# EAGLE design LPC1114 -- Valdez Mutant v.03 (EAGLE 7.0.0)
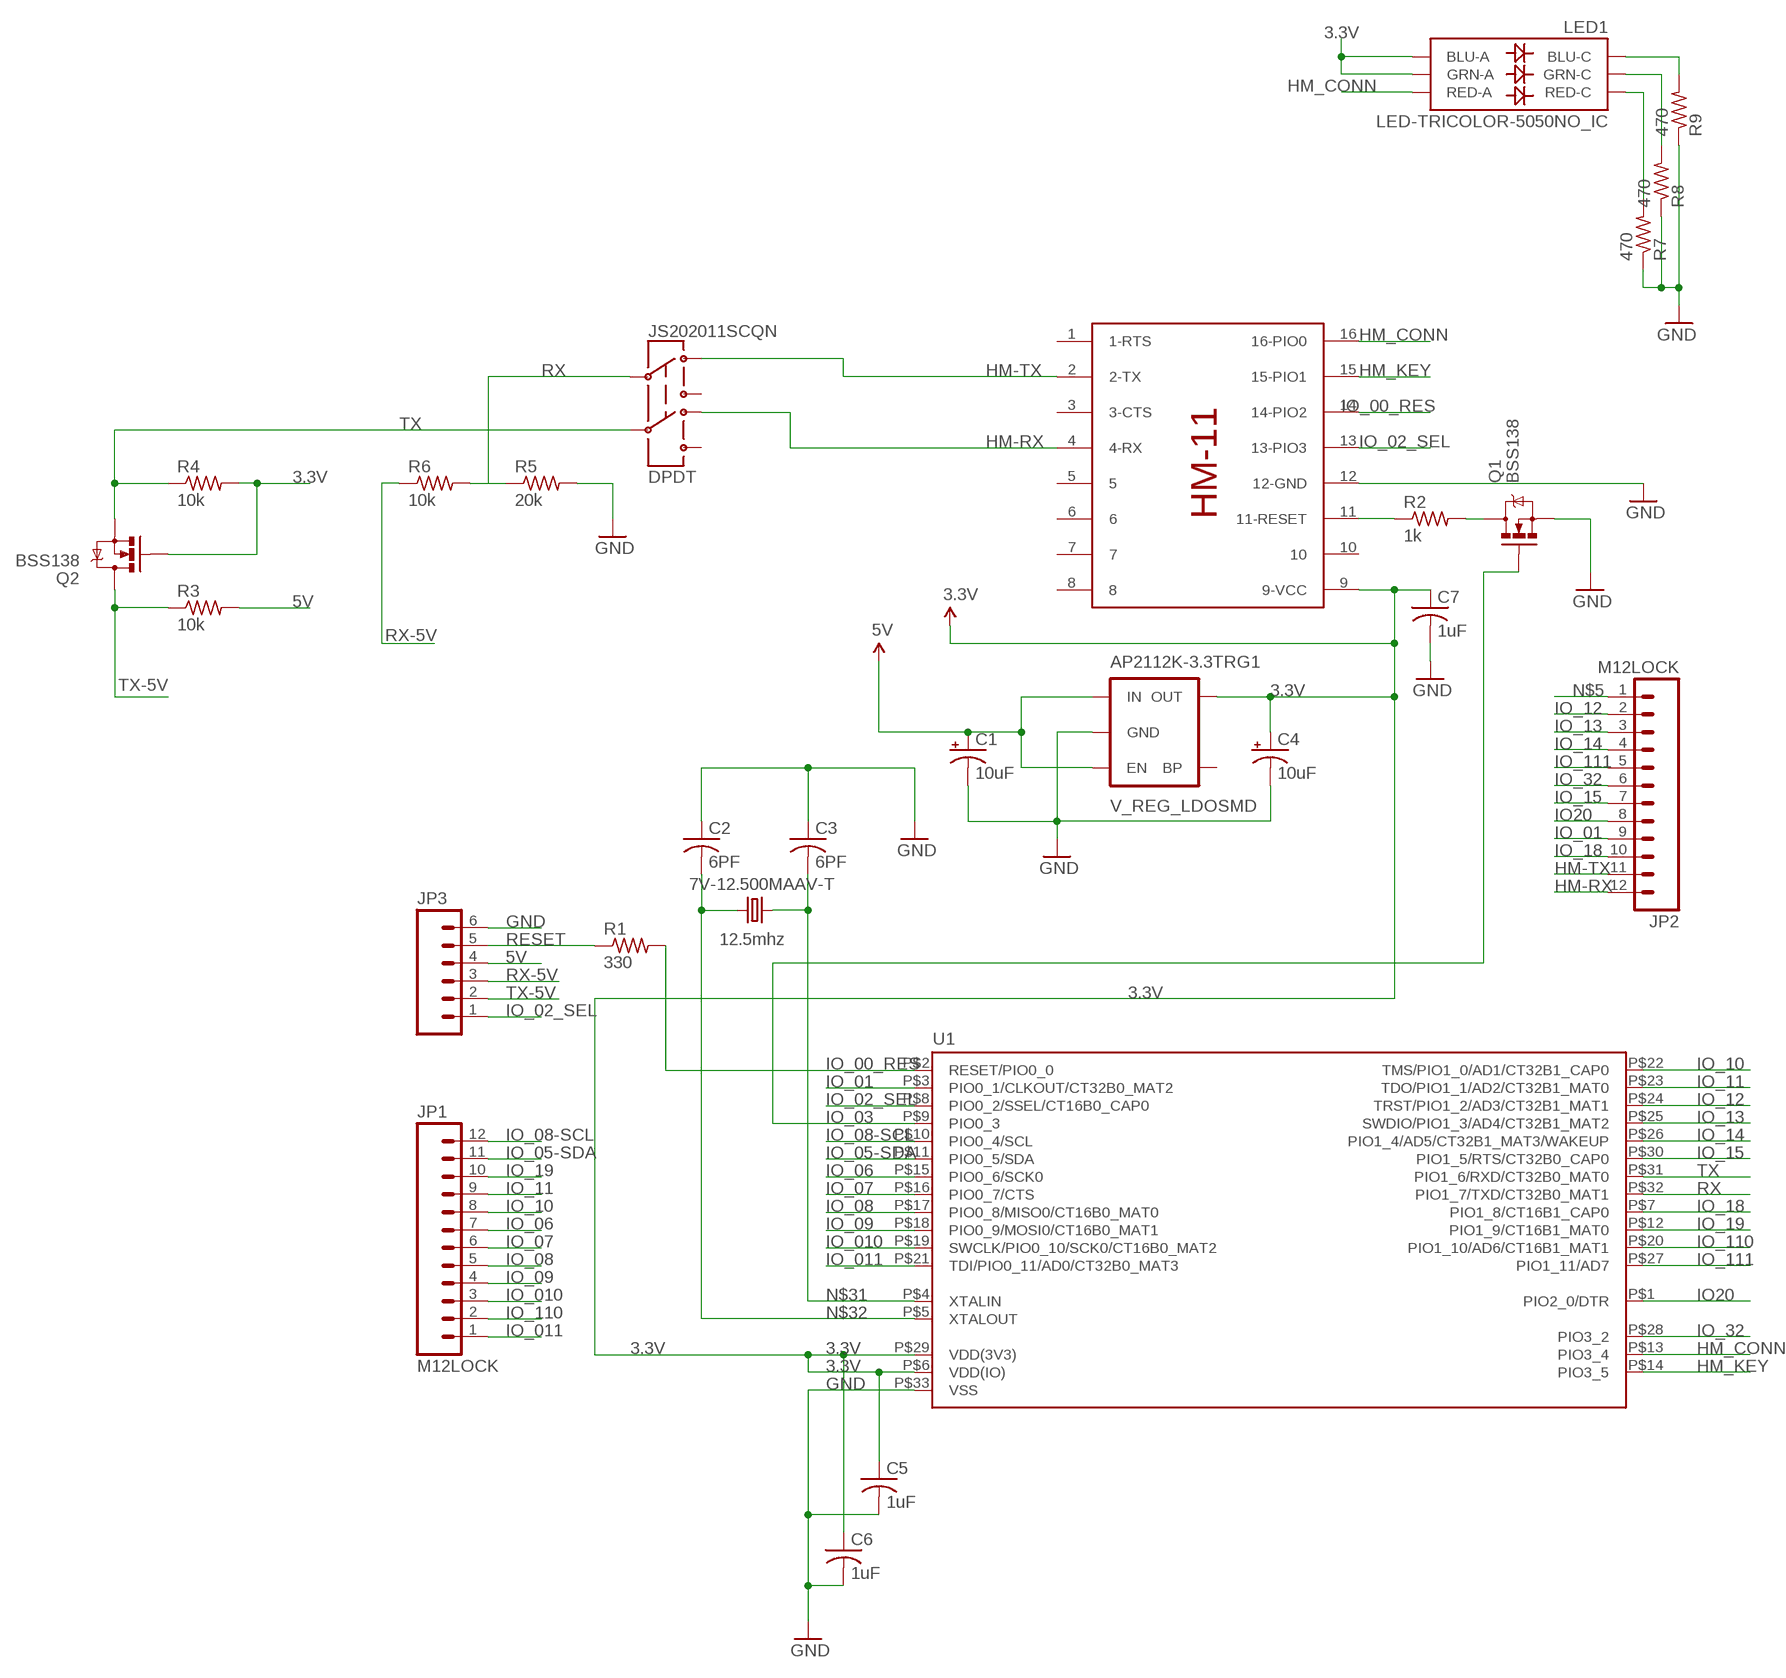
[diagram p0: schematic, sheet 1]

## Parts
7V-12.500MAAV-T  12.5mhz  CRYSTAL5X3  [CRYSTAL-SMD-5X3]
AP2112K-3.3TRG1  V_REG_LDOSMD  [SOT23-5]
C1  10uF  CAP_POL1206  [EIA3216]
C2  6PF  C-USC0402K  [C0402K]
C3  6PF  C-USC0402K  [C0402K]
C4  10uF  CAP_POL1206  [EIA3216]
C5  1uF  C-USC0402K  [C0402K]
C6  1uF  C-USC0402K  [C0402K]
C7  1uF  C-USC0402K  [C0402K]
JP1  M12LOCK  [1X12_LOCK]
JP2  M12LOCK  [1X12_LOCK]
JP3  M06LOCK  [1X06_LOCK]
JS202011SCQN  DPDT  SWITCH-DPDTAYZ0202  [AYZ0202]
LED1  LED-TRICOLOR-5050NO_IC  [LED-TRICOLOR-5050]
Q1  BSS138  MOSFET-NCHANNELBSS138  [SOT23]
Q2  BSS138  MOSFET-NCHANNELBSS138  [SOT23]
R1  330  R-US_R0402  [R0402]
R2  1k  R-US_R0402  [R0402]
R3  10k  R-US_R0402  [R0402]
R4  10k  R-US_R0402  [R0402]
R5  20k  R-US_R0402  [R0402]
R6  10k  R-US_R0402  [R0402]
R7  470  R-US_R0402  [R0402]
R8  470  R-US_R0402  [R0402]
R9  470  R-US_R0402  [R0402]
U1  LPC1113/4_QFN  [HVQFN33-7X7]
U$1  HM-11  [HM-11]

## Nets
3.3V: AP2112K-3.3TRG1.5(OUT) C4.A(+) C5.1 C6.1 C7.1 LED1.1(GRN-A) LED1.3(BLU-A) Q2.1(G) R4.2 U1.P$6(VDD(IO)) U1.P$29(VDD(3V3)) U$1.9(9-VCC)
5V: AP2112K-3.3TRG1.1(IN) AP2112K-3.3TRG1.3(EN) C1.A(+) JP3.4 R3.2
GND: AP2112K-3.3TRG1.2(GND) C1.C(-) C2.1 C3.1 C4.C(-) C5.2 C6.2 C7.2 JP3.6 Q1.2(S) R5.2 R7.1 R8.1 R9.1 U1.P$33(VSS) U$1.12(12-GND)
HM-RX: JP2.12 JS202011SCQN.4 U$1.4(4-RX)
HM-TX: JP2.11 JS202011SCQN.1 U$1.2(2-TX)
HM_CONN: LED1.2(RED-A) U1.P$13(PIO3_4) U$1.16(16-PIO0)
HM_KEY: U1.P$14(PIO3_5) U$1.15(15-PIO1)
IO20: JP2.8 U1.P$1(PIO2_0/DTR)
IO_00_RES: R1.2 U1.P$2(RESET/PIO0_0) U$1.14(14-PIO2)
IO_01: JP2.9 U1.P$3(PIO0_1/CLKOUT/CT32B0_MAT2)
IO_02_SEL: JP3.1 U1.P$8(PIO0_2/SSEL/CT16B0_CAP0) U$1.13(13-PIO3)
IO_03: Q1.1(G) U1.P$9(PIO0_3)
IO_05-SDA: JP1.11 U1.P$11(PIO0_5/SDA)
IO_06: JP1.7 U1.P$15(PIO0_6/SCK0)
IO_07: JP1.6 U1.P$16(PIO0_7/CTS)
IO_08: JP1.5 U1.P$17(PIO0_8/MISO0/CT16B0_MAT0)
IO_08-SCL: JP1.12 U1.P$10(PIO0_4/SCL)
IO_09: JP1.4 U1.P$18(PIO0_9/MOSI0/CT16B0_MAT1)
IO_10: JP1.8 U1.P$22(TMS/PIO1_0/AD1/CT32B1_CAP0)
IO_010: JP1.3 U1.P$19(SWCLK/PIO0_10/SCK0/CT16B0_MAT2)
IO_11: JP1.9 U1.P$23(TDO/PIO1_1/AD2/CT32B1_MAT0)
IO_011: JP1.1 U1.P$21(TDI/PIO0_11/AD0/CT32B0_MAT3)
IO_12: JP2.2 U1.P$24(TRST/PIO1_2/AD3/CT32B1_MAT1)
IO_13: JP2.3 U1.P$25(SWDIO/PIO1_3/AD4/CT32B1_MAT2)
IO_14: JP2.4 U1.P$26(PIO1_4/AD5/CT32B1_MAT3/WAKEUP)
IO_15: JP2.7 U1.P$30(PIO1_5/RTS/CT32B0_CAP0)
IO_18: JP2.10 U1.P$7(PIO1_8/CT16B1_CAP0)
IO_19: JP1.10 U1.P$12(PIO1_9/CT16B1_MAT0)
IO_32: JP2.6 U1.P$28(PIO3_2)
IO_110: JP1.2 U1.P$20(PIO1_10/AD6/CT16B1_MAT1)
IO_111: JP2.5 U1.P$27(PIO1_11/AD7)
N$2: LED1.4(BLU-C) R9.2
N$3: LED1.6(GRN-C) R8.2
N$4: LED1.5(RED-C) R7.2
N$5: JP2.1
N$8: Q1.3(D) R2.2
N$9: R2.1 U$1.11(11-RESET)
N$31: 7V-12.500MAAV-T.3 C3.2 U1.P$4(XTALIN)
N$32: 7V-12.500MAAV-T.1 C2.2 U1.P$5(XTALOUT)
RESET: JP3.5 R1.1
RX: JS202011SCQN.2 R5.1 R6.2 U1.P$32(PIO1_7/TXD/CT32B0_MAT1)
RX-5V: JP3.3 R6.1
TX: JS202011SCQN.5 Q2.2(S) R4.1 U1.P$31(PIO1_6/RXD/CT32B0_MAT0)
TX-5V: JP3.2 Q2.3(D) R3.1
Unconnected: AP2112K-3.3TRG1.4(BP) JS202011SCQN.3 JS202011SCQN.6 U$1.1(1-RTS) U$1.3(3-CTS) U$1.5 U$1.6 U$1.7 U$1.8 U$1.10

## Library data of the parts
7V-12.500MAAV-T = SparkFun-FreqCtrl:CRYSTAL: Various standard crystals. Proven footprints. Spark Fun Electronics SKU : COM-00534
AP2112K-3.3TRG1 = SparkFun-PowerIC:V_REG_LDO: Voltage Regulator LDO Standard 150mA LDO voltage regulator in SOT-23 layout. Micrel part MIC5205. BP (by-pass) pin is used to lower output noise with 470pF cap.
C1 C4 = SparkFun-Capacitors:CAP_POL: Capacitor Polarized
C2 C3 C5-C7 = resistor:C-US: CAPACITOR, American symbol
JP1 JP2 = SparkFun-Connectors:M12: Header 12 Standard 12-pin 0.1" header. Use with straight break away headers (SKU : PRT-00116), right angle break away headers (PRT-00553), swiss pins (PRT-00743), machine pins (PRT-00117), and female headers (PRT-00115).
JP3 = SparkFun-Connectors:M06: Header 6 Standard 6-pin 0.1" header. Use with straight break away headers (SKU : PRT-00116), right angle break away headers (PRT-00553), swiss pins (PRT-00743), machine pins (PRT-00117), and female headers (PRT-00115). Molex polarized connector foot print use with SKU : PRT-08094 with associated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
JS202011SCQN = SparkFun-Electromechanical:SWITCH-DPDT: DPDT Version of the COM-00597; PROD_ID: SWCH-08179
LED1 = SparkFun-LED:LED-TRICOLOR-5050
Q1 Q2 = SparkFun-DiscreteSemi:MOSFET-NCHANNEL: Common NMOSFET Parts MFG P/NStore IDProd ID FDD8780TRANS-09984 SI7820DNTRANS-11055 FDS6630AIC-08089 2N7002PWTRANS-11151 FQP30N06L COM-10213TRANS-10060 BSS123LT1GTRANS-08345 BSS138TRANS-00830 BS170 2N7000; PROD_ID: TRANS-00830
R1-R9 = resistor:R-US_: RESISTOR, American symbol
U1 = microbuilder:LPC1113/4_QFN: LPC1113/4 ARM Cortex-M0 processor, running at frequencies of up to 50 MHz. QFN 33 Pin Package; DIGIKEY#: 568-4948-ND; MANF: NXP; MANF#: LPC1114FHN33/301,5
U$1 = HM-11:HM-11

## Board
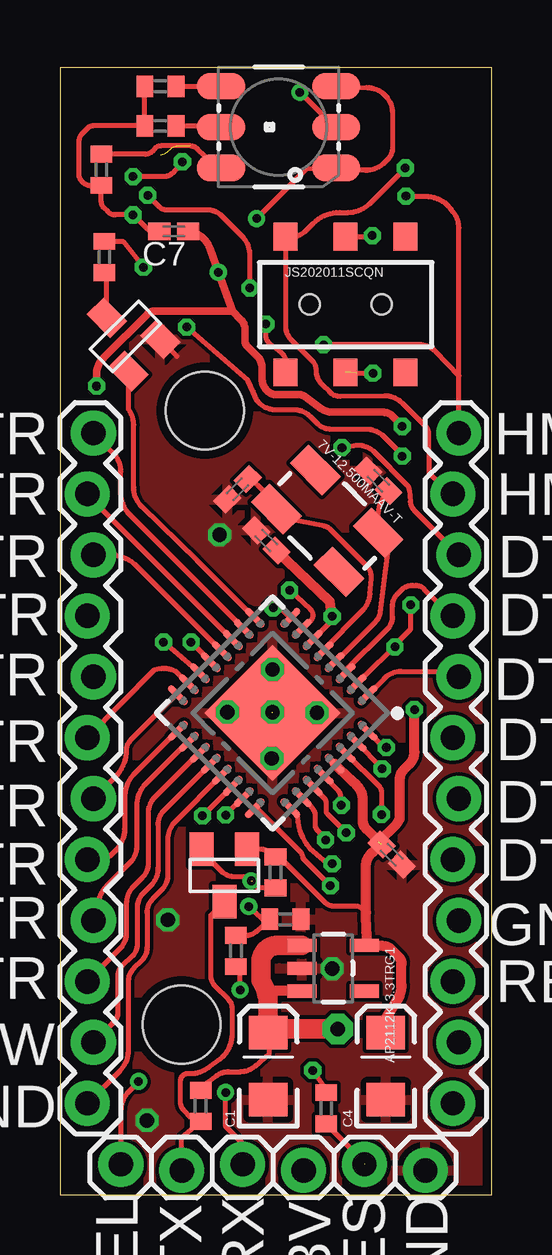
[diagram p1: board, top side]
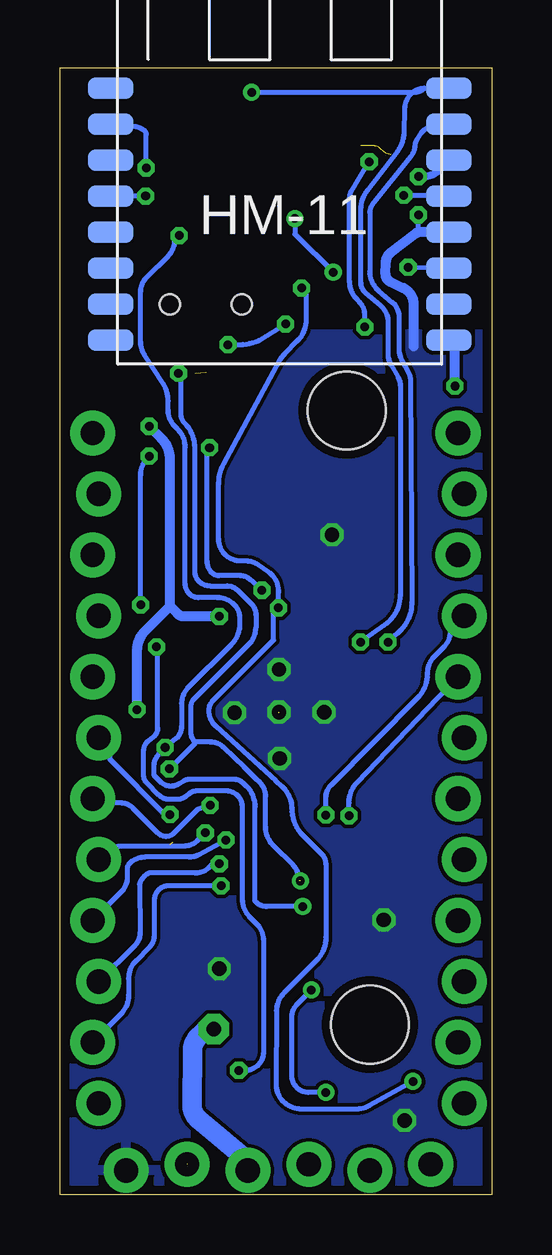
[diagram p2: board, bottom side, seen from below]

Size 18 x 46.97 mm. Coordinates in mm from the lower left corner, seen from the top.
Outline: 0,0 18,0 18,46.97 0,46.97 0,0
Copper layers (1*16): Top 0.0356mm / dielectric 1.5011mm / Bottom 0.0356mm
Design rules "LaenPCBOrder": minimum track width 6mil, minimum drill 13mil, track to track 6mil, track to pad 6mil, pad to pad 6mil, via to via 6mil, smd to smd 6mil, copper to edge 15mil, drill to drill 6mil, minimum pad ring 7mil, minimum via ring 7mil, stop-mask expansion 3mil, vias tented up to drill 0mil, thermal gap 10mil
Holes 3.25 mm at 5.07,7.1 6.04,32.68

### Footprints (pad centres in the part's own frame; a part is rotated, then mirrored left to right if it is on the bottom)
CRYSTAL-SMD-5X3 = smd 1.9 x 1.1: 1 -1.85,-1.15; 2 1.85,-1.15; 3 1.85,1.15; 4 -1.85,1.15
SOT23-5 = smd 0.55 x 1.2: 1 -0.95,-1.3; 2 0,-1.3; 3 0.95,-1.3; 4 0.95,1.3; 5 -0.95,1.3
EIA3216 = smd 1.4 x 1.6: A 1.4,0; C -1.4,0
C0402K = smd 0.925 x 0.74: 1 -0.6,0; 2 0.6,0
1X12_LOCK = drill 1.016 pad 1.88: 1 0,0.127; 2 2.54,-0.127; 3 5.08,0.127; 4 7.62,-0.127; 5 10.16,0.127; 6 12.7,-0.127; 7 15.24,0.127; 8 17.78,-0.127; 9 20.32,0.127; 10 22.86,-0.127; 11 25.4,0.127; 12 27.94,-0.127
1X06_LOCK = drill 1.016 pad 1.88: 1 0,0; 2 2.54,-0.254; 3 5.08,0; 4 7.62,-0.254; 5 10.16,0; 6 12.7,-0.254
AYZ0202 = smd 1 x 1.15: 1 -2.5,2.825; 2 0,2.825; 3 2.5,2.825; 4 -2.5,-2.825; 5 0,-2.825; 6 2.5,-2.825 | hole 0.85: 1.5,0; -1.5,0
LED-TRICOLOR-5050 = smd 2 x 1.1: 1 -2.4,1.7; 2 -2.4,0; 3 -2.4,-1.7; 4 2.4,-1.7; 5 2.4,0; 6 2.4,1.7
SOT23 = smd 1 x 1.4: 1 -0.95,-1.1; 2 0.95,-1.1; 3 0,1.1
R0402 = smd 0.7 x 0.9: 1 -0.65,0; 2 0.65,0
HVQFN33-7X7 = smd 1.067 x 0.3: P$1 -3.327,2.275; P$2 -3.327,1.625; P$3 -3.327,0.975; P$4 -3.327,0.325; P$5 -3.327,-0.325; P$6 -3.327,-0.975; P$7 -3.327,-1.625; P$8 -3.327,-2.275; P$17 3.327,-2.275; P$18 3.327,-1.625; P$19 3.327,-0.975; P$20 3.327,-0.325; P$21 3.327,0.325; P$22 3.327,0.975; P$23 3.327,1.625; P$24 3.327,2.275 | smd 0.3 x 1.067: P$9 -2.275,-3.327; P$10 -1.625,-3.327; P$11 -0.975,-3.327; P$12 -0.325,-3.327; P$13 0.325,-3.327; P$14 0.975,-3.327; P$15 1.625,-3.327; P$16 2.275,-3.327; P$25 2.275,3.327; P$26 1.625,3.327; P$27 0.975,3.327; P$28 0.325,3.327; P$29 -0.325,3.327; P$30 -0.975,3.327; P$31 -1.625,3.327; P$32 -2.275,3.327 | smd 4 x 4: P$33 0,0
HM-11 = smd 1.9 x 0.9: 1 -0.3,11.5; 2 -0.3,10; 3 -0.3,8.5; 4 -0.3,7; 5 -0.3,5.5; 6 -0.3,4; 7 -0.3,2.5; 8 -0.3,1; 9 13.8,1; 10 13.8,2.5; 11 13.8,4; 12 13.8,5.5; 13 13.8,7; 14 13.8,8.5; 15 13.8,10; 16 13.8,11.5

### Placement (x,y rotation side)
7V-12.500MAAV-T  11.15,28.09 315 top
AP2112K-3.3TRG1  11.4,9.44 270 top
C1  8.69,5.36 90 top
C2  7.4,29.41 45 top
C3  13.28,29.75 315 top
C4  13.59,5.36 90 top
C5  13.84,14.18 315 top
C6  8.61,27.27 135 top
C7  4.75,40.16 180 top
JP1  1.27,3.81 90 top
JP2  16.51,3.81 90 top
JP3  2.54,1.27 0 top
JS202011SCQN  11.91,37.11 0 top
LED1  9.12,44.5 180 top
Q1  2.73,35.78 45 top
Q2  6.86,13.31 180 top
R1  11.1,3.61 90 top
R2  1.85,39.09 270 top
R3  5.87,3.71 90 top
R4  8.99,13.44 90 top
R5  9.4,11.48 0 top
R6  7.34,10.16 90 top
R7  4.19,44.55 0 top
R8  1.73,42.72 90 top
R9  4.19,46.2 0 top
U1  8.87,20.08 225 top
U$1  15.59,34.62 0 bottom

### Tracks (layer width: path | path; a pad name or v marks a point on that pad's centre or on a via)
3.3V  (via drill 0.36, 0.36 pad 0.25)  (1 unrouted)
  Top 0.203: AP2112K-3.3TRG1.5 | 11.35,23.94 U1.P$6 | Q2.1 8.33,14.41 arc-45 8.91,14.17 R4.2 9.15,14.09 11.08,12.16 arc45 11.37,12.04 12.3,12.04 arc-45 12.62,11.9 12.77,11.76 | LED1.3 12.79,46.15 arc-90 13.87,45.07 13.87,43.64 arc-45 13.67,43.16 13.53,43.02 arc-45 12.75,42.7 12.08,42.7 LED1.1 10.26,42.75 v8.2,40.69 | v6.6,38.46 6.6,38.44 6.62,38.42
  Top 0.305: v14.28,32.03 13.86,32.46 arc46 13.5,32.61 11.37,32.61 arc-37 10.88,32.78 10.21,33.27 arc37 9.98,33.35 9,33.35 arc-45 8.68,33.48 8.64,33.52 arc-45 8.43,34.02 8.43,34.44 arc45 8.22,34.96 7.81,35.37 arc-45 7.72,35.58 7.72,36.06 arc45 7.55,36.46 7.19,36.83 | v1.52,33.71 1.52,34.16 arc-45 1.83,34.91 3.62,36.7 arc-45 3.95,36.83 7.19,36.83 | 7.19,36.83 6.62,38.42 6.27,39.43 arc64 C7.1
  Top 0.406: U1.P$29 12.14,17.3 12.38,17.05 arc-45 12.62,16.48 12.62,15.6 arc45 12.77,15.24 C5.1 13.01,14.25 12.98,14.22 arc45 12.75,13.68 12.77,11.76 12.78,10.95 12.78,10.47 AP2112K-3.3TRG1.5 12.73,10.36 13.48,10.36 arc-45 13.84,10.22 14.11,9.95 arc-45 14.25,9.61 14.25,8.75 arc-31 14.07,8.12 13.61,7.37 C4.A | v14.78,20.22 14.78,18.45 arc-45 14.58,17.95 14.34,17.72 arc45 14.17,17.31 14.17,15.78 arc-45 14.04,15.47 13.28,14.71 | 11.35,23.94 v11.35,24.11 11.25,24.73 C6.1
  Bottom 0.203: v8.2,40.69 8.2,40.02 8.17,40.02 v6.6,38.46
  Bottom 0.406: v14.78,20.22 14.78,22.67 arc45 14.43,23.52 13.41,24.54 | 13.41,24.54 13.41,30.67 arc-45 13.76,31.52 v14.28,32.03 | v1.52,33.71 1.52,35.36 U$1.9 | 11.23,23.98 v11.35,24.11 12.81,24.11 arc45 13.1,24.23 13.41,24.54
5V  (via drill 0.6 pad 1.27)
  Top 0.203: AP2112K-3.3TRG1.3 | 8.84,6.91 C1.A 8.74,6.71 8.74,5.89 8.13,5.36 arc-41 7.53,5.13 7.05,5.13 arc37 6.53,4.96 5.93,4.51 R3.2
  Top 0.406: 8.59,8.51 9.68,8.51 AP2112K-3.3TRG1.3
  Top 0.813: 8.77,6.68 C1.A 8.69,8.1 arc17 8.66,8.25 8.59,8.51 8.38,8.94 8.38,9.68 arc-45 8.6,10.2 arc-45 9.06,10.39 AP2112K-3.3TRG1.1 | v11.58,6.91 8.84,6.91
  Bottom 0.813: JP3.4 10.16,1.42 12.18,3.09 arc51 12.49,3.76 12.47,5.97 arc45 12.2,6.62 11.91,6.91 v11.58,6.91
GND  (via drill 0.36, 0.6 pad 0.81)  (1 unrouted)
  Top 0.203: 4.15,40.11 C7.2 3.94,40.16 arc-45 3.58,40.31 v3.05,40.84 2.31,40.84 arc-45 2.01,40.97 1.83,41.15 arc-45 1.73,41.39 R8.1 1.72,42.06 1.3,42.06 arc-45 0.94,42.21 0.9,42.25 arc-45 0.79,42.53 0.79,43.87 arc-45 0.94,44.25 1.16,44.47 arc-45 1.37,44.55 R7.1 | Q1.2 4.18,35.64 4.88,34.95 | 3.54,44.53 R7.1 | R7.1 R9.1
  Bottom 0.203: 3.06,40.12 3.06,40.42 v3.05,40.84
  Bottom 0.406: 3.25,35.36 3.25,37.13 arc-64 3.67,37.79 4.23,38.06 arc64 4.42,38.36 4.41,38.88 arc51 4.21,39.26 3.17,40.07 arc25 3.06,40.12 U$1.12
  other vias: 8.86,20.12 8.86,21.89 10.72,20.09 8.84,18.19 6.99,20.12 3.63,3.1 11.35,9.42 4.5,11.46 6.65,27.51
  pour Bottom: 0,35.86 0,0 17.78,0 17.78,35.86
  pour Top: 0.2,36.07 0,0 17.78,0 17.98,36.07
HM-RX  (via drill 0.36, 0.36 pad 0.25)
  Top 0.203: JS202011SCQN.4 9.41,34.72 arc52 9.22,35.11 8.72,35.51 arc-18 8.66,35.57 8.66,35.57 arc-34 8.59,35.82 v8.59,36.3 | JP2.12 16.64,34.14 | 16.64,34.14 16.64,40.3 arc38 16.41,40.95 16.3,41.09 arc52 15.25,41.6 14.45,41.6 v14.43,41.63 | 16.64,34.14 15.68,35.14 arc46 14.98,35.43 v11,35.43
  Bottom 0.203: v14.43,41.63 15.88,41.63 U$1.4 | v11,35.43 10.5,35.43 arc-25 9.7,35.61 v8.59,36.3
HM-TX  (via drill 0.36 pad 0.25)
  Top 0.203: v14.4,42.8 12.92,41.32 arc-45 12.02,40.95 11.66,40.95 arc45 10.57,40.49 10.27,40.19 arc-45 9.65,39.93 JS202011SCQN.1 9.42,39.92 9.42,36.17 arc45 9.64,35.65 10.52,34.77 arc-45 10.69,34.35 arc45 10.93,33.77 11.25,33.45 arc46 11.68,33.28 13.54,33.3 arc-45 14.28,33 15.25,32.05 arc-45 15.37,31.76 15.39,30.07 JP2.11
  Bottom 0.203: v14.4,42.8 14.4,44.2 arc-45 14.45,44.32 arc-45 14.94,44.53 15.79,44.53 U$1.2
HM_CONN  (via drill 0.36, 0.36 pad 0.25)
  Top 0.203: U1.P$13 6.22,22.2 6.22,22.28 v5.46,23.04 | LED1.2 11.51,44.45 v10.01,45.95
  Bottom 0.203: 2.81,46.12 arc-54 3.43,45.81 arc-34 3.62,45.27 3.65,44.26 arc36 3.91,43.51 5.18,41.86 arc-37 5.46,41.09 5.46,38.03 arc-50 5.26,37.6 4.64,37.08 arc50 4.32,36.38 4.32,35.03 arc-30 4.21,34.6 3.89,34.06 arc30 3.81,33.74 3.81,25.02 arc55 4.47,23.74 v5.46,23.04 | 2.81,46.12 U$1.16 | v10.01,45.95 3.24,45.95 arc-45 2.81,46.12
HM_KEY  (via drill 0.36 pad 0.25)
  Top 0.203: U1.P$14 5.83,21.76 v4.32,23.04
  Bottom 0.203: U$1.15 1.86,44.55 2.34,44.55 arc-57 2.96,44.22 3.1,44 arc-30 3.18,43.76 arc35 3.37,43.27 4.97,41.26 arc-39 5.08,40.95 5.08,38.48 arc-49 4.71,37.69 4.13,37.19 arc49 3.86,36.6 3.86,35.25 arc-28 3.74,34.78 3.46,34.26 arc28 3.38,33.95 3.33,24.67 arc48 3.88,23.43 v4.32,23.04
IO20
  Top 0.203: U1.P$1 13.53,21.53 arc-45 14.23,21.82 16.41,21.82 JP2.8
IO_00_RES  (via drill 0.36, 0.36 pad 0.25)
  Top 0.203: 12.37,21.31 U1.P$2 13.11,22.02 v13.97,22.84 13.97,22.91 14.59,23.53 arc45 14.63,23.62 v14.63,24.59 | v14.28,30.79 14.22,30.89 13.5,31.61 arc45 12.79,31.9 11.33,31.9 arc-45 10.72,32.16 10.45,32.43 arc45 9.76,32.72 8.95,32.72 arc-48 8.22,33.1 8.05,33.49 7.84,33.94 v5.28,36.17 5.54,36.17 | v5.11,43.05 4.69,42.58 arc-44 4.35,42.44 v3.05,42.44 | 11.19,4.31 R1.2 11.1,4.42 v10.54,5.18
  Bottom 0.203: v13.97,22.84 13.92,22.78 13.92,19.44 arc52 14.09,19.09 14.33,18.91 arc-52 14.5,18.55 14.5,17.43 arc-45 14.41,17.2 13.86,16.65 arc-45 13.46,16.48 13.09,16.48 arc-41 12.72,16.62 12.64,16.69 arc41 12.25,16.84 11.09,16.84 arc49 10.56,16.6 arc41 10.39,16.15 10.39,12.32 arc-45 10.08,11.58 9.8,11.3 arc45 9.5,10.58 9.5,5.94 arc54 9.81,5.34 arc36 10.31,5.18 v10.54,5.18 | v14.63,24.59 14.63,30.01 arc49 v14.28,30.79 | v5.28,36.17 5.28,36.66 arc-45 5.51,37.21 5.6,37.3 arc45 5.92,38.06 5.92,41.56 arc27 5.85,41.83 v5.11,43.05
  Bottom 0.305: v3.05,42.44 2.82,42.44 arc-45 2.22,42.69 U$1.14
IO_01
  Top 0.203: U1.P$3 11.91,21.84 13.68,23.61 arc45 13.87,24.07 13.87,24.52 arc-45 14.1,25.07 14.23,25.21 arc-45 14.7,25.4 14.83,25.4 arc-45 15.19,25.25 15.65,24.79 16.26,24.21 JP2.9
IO_02_SEL  (via drill 0.36, 0.36 pad 0.25)
  Top 0.203: v8.89,24.46 9.3,24.36 U1.P$8 | v7.92,37.8 7.92,39.14 arc45 7.59,39.96 6.74,40.81 arc45 6.16,41.05 4.47,41.05 arc-45 4.12,41.19 v3.66,41.66 | v3.28,4.72 3.28,4.7 2.87,4.29 arc45 2.54,3.5 JP3.1
  Bottom 0.203: v3.28,4.72 5.08,3.72 arc29 5.62,3.58 7.94,3.58 arc45 8.69,3.89 arc45 8.99,4.61 8.97,7.67 arc45 8.66,8.4 7.32,9.75 arc-45 6.91,10.74 6.91,13.78 arc-45 7.08,14.19 7.87,14.98 arc45 8.33,16.09 arc-49 8.76,17.04 8.99,17.25 11.5,19.52 arc48 11.79,20.18 arc45 11.61,20.59 9.09,23.11 9.09,24.28 v8.89,24.46 8.88,25.12 arc-56 9.31,25.96 9.72,26.25 arc-35 10.24,26.42 10.47,26.42 arc90 11.38,27.33 11.38,29.63 arc28 11.17,30.46 8.81,34.81 arc17 8.62,35.06 8.09,35.6 arc-45 7.72,36.48 7.72,37.59 v7.92,37.8 | v3.66,41.66 1.82,41.66 U$1.13
IO_03
  Top 0.203: U1.P$9 8.11,24.04 5.71,26.44 3.42,28.67 arc-46 3.07,29.49 3.07,32.1 arc36 2.88,32.71 arc-36 2.87,32.73 2.87,33.84 Q1.1
IO_05-SDA
  Top 0.203: JP1.11 1.14,29.19 U1.P$11
IO_06
  Top 0.203: U1.P$15 5.31,21.36 4.83,21.81 arc45 3.94,21.87 JP1.7
IO_07
  Top 0.203: U1.P$16 4.82,20.82 2.94,18.94 arc45 2.77,18.53 arc-45 2.31,17.42 JP1.6
IO_08
  Top 0.203: U1.P$17 4.88,19.34 3.13,17.58 arc45 2.69,16.52 2.69,15.23 arc-45 2.34,14.38 2.13,14.17 arc-45 1.47,13.89 1.22,13.89 JP1.5
IO_08-SCL
  Top 0.203: U1.P$10 7.67,23.6 2.91,28.36 arc-45 2.54,29.25 2.54,30.13 arc45 2.2,30.94 JP1.12
IO_09
  Top 0.203: U1.P$18 5.31,18.88 3.59,17.15 arc45 3.2,16.22 3.2,14.5 arc-45 2.93,13.85 1.93,12.85 arc45 1.57,12 1.57,11.61 JP1.4
IO_10  (via drill 0.36 pad 0.25)
  Top 0.203: U1.P$22 v5.94,15.8
  Bottom 0.203: v5.94,15.8 5.94,16.35 arc44 5.6,17.2 JP1.8
IO_010
  Top 0.203: U1.P$19 5.79,18.42 3.96,16.59 arc45 3.68,15.91 3.68,13.83 arc-45 3.42,13.2 3.06,12.84 arc45 2.77,12.14 2.77,10.93 arc-45 2.48,10.22 JP1.3
IO_11  (via drill 0.36 pad 0.25)
  Top 0.203: U1.P$23 7.61,16.58 v6.91,15.82
  Bottom 0.203: v6.91,15.82 6.91,16.55 arc45 6.69,17.09 3.06,20.73 arc-45 2.67,21.7 2.67,21.75 arc45 2.39,22.43 2.01,22.81 arc-45 1.7,23.55 1.7,23.57 JP1.9
IO_011
  Top 0.203: U1.P$21 4.8,15.55 arc45 4.5,14.81 4.5,13.34 arc-45 4.22,12.68 3.87,12.32 arc45 3.63,11.76 3.63,10.3 arc-45 3.4,9.76 3.08,9.43 arc45 2.85,8.87 2.85,6.02 arc-45 2.49,5.15 JP1.1
IO_12  (via drill 0.36 pad 0.25)
  Top 0.203: U1.P$24 8.19,16.12 10.03,14.28 arc-45 10.13,14.02 v11.28,12.88
  Bottom 0.203: v11.28,12.88 13.49,12.88 arc-45 13.88,12.72 arc-45 14.07,12.25 14.07,10.78 arc45 14.26,10.33 14.83,9.75 arc-45 15.14,9.02 15.14,8.32 arc45 15.47,7.51 JP2.2
IO_13  (via drill 0.36 pad 0.25)
  Top 0.203: U1.P$25 9.87,15.81 9.91,15.71 arc40 10.4,14.46 11.15,13.82 v11.35,13.79
  Bottom 0.203: v11.35,13.79 11.43,13.99 11.78,13.64 arc45 12.35,13.41 14.3,13.41 arc-45 14.68,12.95 14.66,10.92 arc46 14.87,10.4 JP2.3
IO_14  (via drill 0.36 pad 0.25)
  Top 0.203: U1.P$26 10.12,16.58 10.54,16.09 arc-41 10.64,15.82 10.64,15.43 arc40 10.73,15.18 v11.07,14.78
  Bottom 0.203: v11.07,14.78 12.22,14.17 arc28 12.6,14.07 14.46,14.07 arc-45 15.1,13.8 arc-45 15.19,13.59 15.19,13.24 arc45 15.45,12.62 JP2.4
IO_15  (via drill 0.36 pad 0.25)
  Top 0.203: U1.P$30 13.31,17.01 arc-45 13.41,16.78 v13.41,15.85
  Bottom 0.203: v13.41,15.85 13.56,15.8 15.92,18.16 arc57 15.93,18.16 arc-57 16.1,18.77 JP2.7
IO_18  (via drill 0.36 pad 0.25)
  Top 0.203: U1.P$7 10.05,23.54 10.45,23.92 arc94 10.45,24.4 v9.58,25.2 | v11.76,31.14 12.24,31.23 arc-55 13.12,30.95 14.46,29.61 arc-40 14.57,29.38 14.61,28.87 arc40 14.77,28.54 JP2.10
  Bottom 0.203: v9.58,25.2 10.1,25.66 arc-42 10.48,25.81 11.38,25.81 arc47 11.68,25.94 arc43 11.86,26.41 11.86,31.04 v11.76,31.14
IO_19
  Top 0.203: JP1.10 2.07,26.67 arc-45 3.22,26.19 U1.P$12
IO_32  (via drill 0.36 pad 0.25)
  Top 0.203: U1.P$28 10.99,17.48 11.6,16.85 arc-44 11.71,16.58 11.71,16.36 v11.73,16.23
  Bottom 0.203: v11.73,16.23 12.27,16.05 13.25,15.07 arc45 13.58,14.94 arc45 13.9,15.07 14.94,16.11 arc-45 15.48,16.33 16.46,16.33 JP2.6
IO_110
  Top 0.203: U1.P$20 6.28,17.96 4.34,16.03 arc45 4.09,15.41 4.09,13.62 arc-45 3.78,12.88 3.46,12.56 arc45 3.23,11.98 3.23,10.44 arc-45 3.03,9.96 2.58,9.51 arc45 2.41,9.12 2.41,7.56 arc-45 2.27,7.23 JP1.2
IO_111  (via drill 0.36 pad 0.25)
  Top 0.203: U1.P$27 10.53,17.03 11.02,16.54 arc-45 11.1,16.34 11.1,16.01 arc45 11.16,15.87 v11.94,15.09
  Bottom 0.203: v11.94,15.09 12.25,14.78 arc45 12.85,14.53 15.39,14.53 arc-45 16.13,14.22 JP2.5
N$2
  Top 0.203: R9.2 6.49,46.2 LED1.4
N$3  (4 unrouted)
  Top 0.203: LED1.6 6.68,42.7 5.72,43.61 arc44 5.45,43.72 4.21,43.72 arc45 3.97,43.62 3.84,43.48 arc-45 3.56,43.37 R8.2
N$4
  Top 0.203: R7.2 7.02,44.55 LED1.5
N$8
  Top 0.203: Q1.3 1.96,38.34 R2.2
N$9  (via drill 0.36 pad 0.25)
  Top 0.203: R2.1 2.63,39.74 v3.48,38.66
  Bottom 0.203: v3.48,38.66 1.8,38.63 U$1.11
N$31
  Top 0.203: U1.P$4 11.48,22.2 13.17,23.89 arc38 13.36,24.29 13.59,26.11 13.69,26.92 7V-12.500MAAV-T.3 13.27,28.29 arc-45 C3.2
N$32
  Top 0.203: U1.P$5 10.99,22.7 12.61,24.34 arc40 12.93,25.05 12.98,25.7 arc49 12.78,26.23 11.29,27.73 arc34 11.03,27.87 9.41,28.19 7V-12.500MAAV-T.1 9.03,28.79 8.26,29.57 7.85,29.88 C2.2
RESET  (1 unrouted)
  Top 0.203: 12.7,1.29 12.7,1.36 R1.1
RX  (via drill 0.36, 0.36 pad 0.25)
  Top 0.203: U1.P$32 12.87,19.34 13.18,18.97 13.51,18.64 v13.61,18.64 | JS202011SCQN.2 12.98,39.93 v13.03,39.98 | R6.2 7.78,10.81 arc42 8.17,10.96 R5.1 8.46,11.48 v7.87,12.01
  Bottom 0.203: v13.03,39.98 13.21,39.8 arc45 13.48,39.15 14.39,38.24 arc-45 14.63,37.66 14.63,35.53 arc-33 14.48,35.03 13.7,33.8 arc33 13.49,33.09 13.49,32.69 arc-45 13.22,32.04 13.08,31.91 arc45 12.78,31.16 12.78,25.45 arc-90 12.22,24.89 11.43,24.89 arc45 10.73,24.6 arc45 10.49,24.02 10.49,23.79 arc45 10.85,22.94 12.67,21.11 arc-45 12.93,20.48 12.93,19.5 arc51 13.16,19.01 v13.61,18.64 13.96,18.24 arc-41 14.07,17.94 14.07,17.48 13.81,17.21 arc-77 13.03,17.13 12.86,17.23 arc32 12.56,17.32 10.74,17.32 arc43 10.39,17.19 10.24,17.04 10.21,17.01 arc45 9.86,16.17 9.86,12.22 arc-45 9.37,12.01 v7.87,12.01
RX-5V  (via drill 0.36)
  Top 0.203: JP3.3 7.62,2.13 6.91,2.85 v6.91,4.27 | v7.52,8.53 7.52,9.33 R6.1
  Bottom 0.203: v6.91,4.27 7.65,4.27 arc45 8.12,4.46 arc45 8.33,4.97 8.33,7.39 arc45 8.1,7.96 v7.52,8.53
TX  (via drill 0.36, 0.36 pad 0.25)  (2 unrouted)
  Top 0.203: U1.P$31 v13.44,17.75 | 12.37,34.24 v13.06,34.24 | Q2.2 5.91,14.31 6.73,13.49 arc45 7.29,13.26 7.8,13.26 v7.98,13.08 8.27,12.79 R4.1
  Bottom 0.203: v13.06,34.24 12.95,33.93 12.95,32.56 arc-45 12.78,32.13 arc45 12.37,31.15 12.37,25.96 arc-45 12.21,25.57 arc-45 11.74,25.38 11.02,25.38 arc45 10.59,25.2 10.02,24.62 arc45 9.83,24.17 9.83,23.63 arc45 10.11,22.97 12.4,20.66 arc-45 12.55,20.32 12.55,19.3 arc-45 U1.P$31 | U1.P$31 11.73,18.87 arc44 11.18,18.65 10.31,17.8 9.78,17.3 9.66,17.18 arc45 9.42,16.61 9.42,15.33 arc-45 9.11,14.57 8.26,13.72 arc45 8.04,13.18 8.04,13.08 | U1.P$31 12.37,18.82 v13.44,17.75
TX-5V
  Top 0.203: JP3.2 5.08,2.4 R3.1 5.48,3.21 5.16,3.53 arc-45 5.03,3.84 5.03,4.75 arc-90 5.33,5.05 5.44,5.05 arc37 6.21,5.31 6.68,5.67 arc53 7.19,6.68 7.19,7.75 arc45 7.03,8.13 6.48,8.69 arc-45 6.3,9.12 6.3,11.65 Q2.3

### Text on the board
tNames: DTR | HM-RX | DTR | HM-TX | DTR | DTR | DTR | DTR | DTR | DTR | DTR | DTR | DTR | DTR | DTR | DTR | DTR | GND | DTR | RESET | RAW | GND | TX | RX | 3.3V | GND | DTR/SEL | CTS/RES

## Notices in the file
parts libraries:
microbuilder: This work is placed in the public domain, and may be freely used for commercial and non-commercial work with the following conditions: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
SparkFun-Connectors: Licensing: Creative Commons ShareAlike 4.0 International - https://creativecommons.org/licenses/by-sa/4.0
